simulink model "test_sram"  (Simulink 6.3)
settings: Solver=ode45  StartTime=0.0  StopTime=200  RelTol=1e-3
undefined symbols (not defined in the file or in its folder): Bit, Location, Lower, netlist, Width
libraries: xbsIndex_r4 x7, adlibrary2 x2, simulink x1, sram_cosim_lib x1

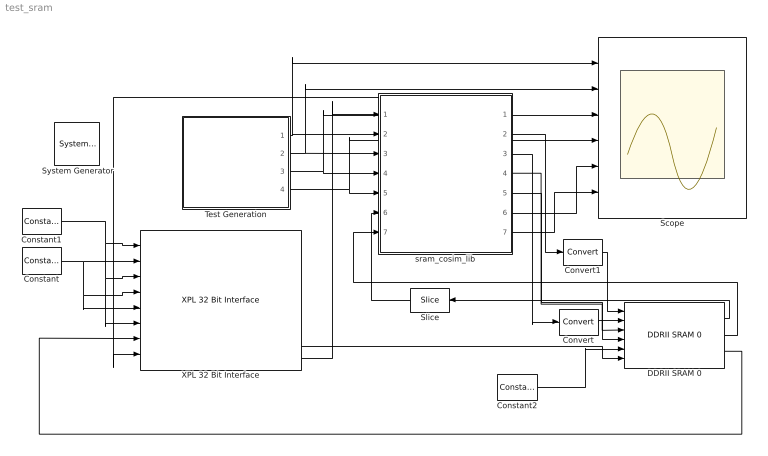
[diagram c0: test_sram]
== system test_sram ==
  " System Generator" : xbsIndex_r4/ System Generator  Tag=genX  xilinxfamily=Virtex2P  part=xc2vp70  speed=-5  package=ff1704  synthesis_tool=XST  directory=./netlist  testbench=off  simulink_period=1  sysclk_period=7.5  incr_netlist=off  trim_vbits=Everywhere in SubSystem  dbl_ovrd=According to Block Masks  core_generation=According to Block Masks  run_coregen=off  deprecated_control=off  eval_field=0  block_type=sysgen
  Constant : xbsIndex_r4/Constant  arith_type=Boolean  const=0  n_bits=16  bin_pt=14  explicit_period=on  period=1  equ=P=C  opselect=C  inp2=PCIN>>17  opr=+  inp1=P  carry=CIN  dbl_ovrd=off  block_type=constant
  Constant1 : xbsIndex_r4/Constant  arith_type=Unsigned  const=0  n_bits=32  bin_pt=0  explicit_period=on  period=1  equ=P=C  opselect=C  inp2=PCIN>>17  opr=+  inp1=P  carry=CIN  dbl_ovrd=off  block_type=constant
  Constant2 : xbsIndex_r4/Constant  arith_type=Unsigned  const=255  n_bits=8  bin_pt=0  explicit_period=on  period=1  equ=P=C  opselect=C  inp2=PCIN>>17  opr=+  inp1=P  carry=CIN  dbl_ovrd=off  block_type=constant
  Convert : xbsIndex_r4/Convert  arith_type=Unsigned  n_bits=21  bin_pt=0  quantization=Truncate  overflow=Wrap  latency=0  dbl_ovrd=off  pipeline=off  block_type=convert
  Convert1 : xbsIndex_r4/Convert  arith_type=Unsigned  n_bits=64  bin_pt=0  quantization=Truncate  overflow=Wrap  latency=0  dbl_ovrd=off  pipeline=off  block_type=convert
  DDRII SRAM 0 : adlibrary2/ADM-XP/DDRII SRAM 0
  Scope : Scope  NumInputPorts=6
  Slice : xbsIndex_r4/Slice  Orientation=left  nbits=16  boolean_output=off  mode=Lower Bit Location + Width  bit1=0  base1=MSB of Input  bit0=0  base0=LSB of Input  dbl_ovrd=off  block_type=slice
  Test Generation : Subsystem
  XPL 32 Bit Interface : adlibrary2/ADM-XPL/XPL 32 Bit Interface  program='load myprogram.txt'  clock_ratio=1.5
  sram_cosim_lib : Subsystem  Tag=configX  BlockChoice=sram_cosim_lib_sim
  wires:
  DDRII SRAM 0/3 -> XPL 32 Bit Interface/7
  Constant/1 -> XPL 32 Bit Interface/5, XPL 32 Bit Interface/4, XPL 32 Bit Interface/2
  Constant1/1 -> XPL 32 Bit Interface/6, XPL 32 Bit Interface/3, XPL 32 Bit Interface/1
  Convert/1 -> DDRII SRAM 0/2
  Convert1/1 -> DDRII SRAM 0/1
  Constant2/1 -> DDRII SRAM 0/5
  XPL 32 Bit Interface/11 -> sram_cosim_lib/1(debug_in)
  sram_cosim_lib/1(debug_out) -> XPL 32 Bit Interface/8
  sram_cosim_lib/2(d_sg) -> Convert1/1
  sram_cosim_lib/3(a_sg) -> Convert/1
  sram_cosim_lib/4(w_sg) -> DDRII SRAM 0/3
  sram_cosim_lib/5(r_sg) -> DDRII SRAM 0/4
  DDRII SRAM 0/1 -> Slice/1
  DDRII SRAM 0/2 -> sram_cosim_lib/7(qv_sg)
  Test Generation/1(d) -> sram_cosim_lib/2(d_sl), Scope/1
  Test Generation/2(a) -> sram_cosim_lib/3(a_sl), Scope/2
  Test Generation/3(w) -> sram_cosim_lib/4(w_sl), Scope/3
  Test Generation/4(r) -> sram_cosim_lib/5(r_sl), Scope/4
  sram_cosim_lib/7(qv_sl) -> Scope/6
  sram_cosim_lib/6(q_sl) -> Scope/5
  Slice/1 -> sram_cosim_lib/6(q_sg)
  XPL 32 Bit Interface/10 -> DDRII SRAM 0/6

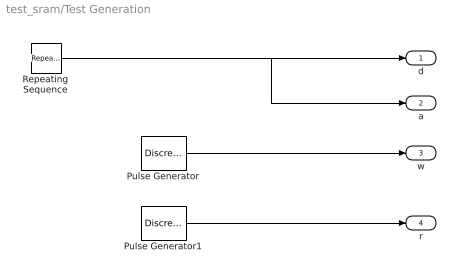
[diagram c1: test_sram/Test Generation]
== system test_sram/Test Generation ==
  Pulse Generator : DiscretePulseGenerator  PulseType=Time based  Period=128  PulseWidth=25
  Pulse Generator1 : DiscretePulseGenerator  PulseType=Time based  Period=128  PulseWidth=25  PhaseDelay=63
  Repeating Sequence : simulink/Sources/Repeating Sequence  rep_seq_t=[1:64]  rep_seq_y=[0:63]
  d : Outport
  a : Outport  Port=2
  w : Outport  Port=3
  r : Outport  Port=4
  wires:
  Repeating Sequence/1 -> d/1, a/1
  Pulse Generator/1 -> w/1
  Pulse Generator1/1 -> r/1

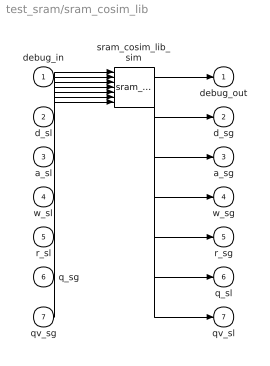
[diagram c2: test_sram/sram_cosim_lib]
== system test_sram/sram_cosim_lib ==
  debug_in : Inport
  d_sl : Inport  Port=2
  a_sl : Inport  Port=3
  w_sl : Inport  Port=4
  r_sl : Inport  Port=5
  q_sg : Inport  Port=6
  qv_sg : Inport  Port=7
  sram_cosim_lib_sim : sram_cosim_lib/sram_cosim_lib_sim
  debug_out : Outport
  d_sg : Outport  Port=2
  a_sg : Outport  Port=3
  w_sg : Outport  Port=4
  r_sg : Outport  Port=5
  q_sl : Outport  Port=6
  qv_sl : Outport  Port=7
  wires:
  debug_in/1 -> sram_cosim_lib_sim/1
  d_sl/1 -> sram_cosim_lib_sim/2
  a_sl/1 -> sram_cosim_lib_sim/3
  w_sl/1 -> sram_cosim_lib_sim/4
  r_sl/1 -> sram_cosim_lib_sim/5
  q_sg/1 -> sram_cosim_lib_sim/6
  qv_sg/1 -> sram_cosim_lib_sim/7
  sram_cosim_lib_sim/1 -> debug_out/1
  sram_cosim_lib_sim/2 -> d_sg/1
  sram_cosim_lib_sim/3 -> a_sg/1
  sram_cosim_lib_sim/4 -> w_sg/1
  sram_cosim_lib_sim/5 -> r_sg/1
  sram_cosim_lib_sim/6 -> q_sl/1
  sram_cosim_lib_sim/7 -> qv_sl/1
